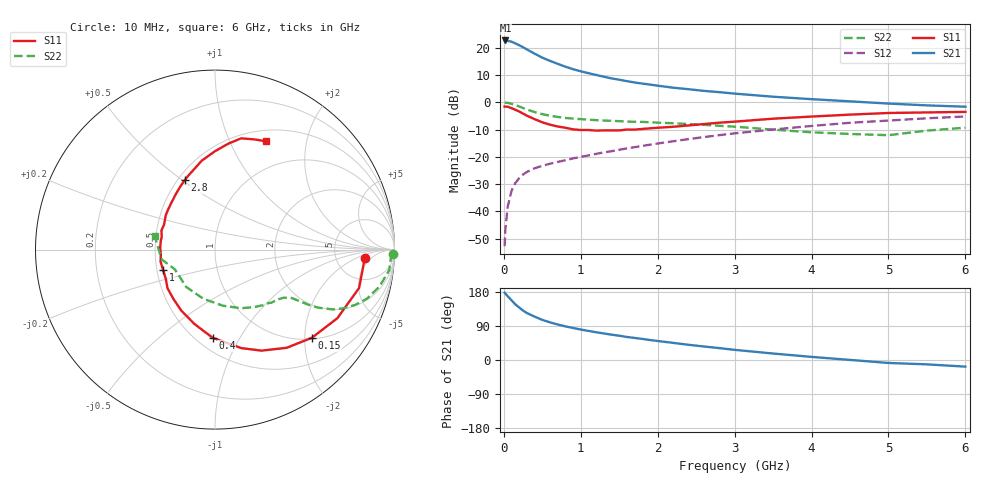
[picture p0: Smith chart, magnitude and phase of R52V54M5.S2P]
! SIEMENS Small Signal Semiconductors
! BFR183
! Si NPN RF Bipolar Junction Transistor in SOT23
! VCE = 2.5 V  IC = 4.5 mA
! Common Emitter S-Parameters:  May  1996
# GHz  S  MA  R  50
!  f  S11  S21  S12  S22
! GHz  MAG  ANG  MAG  ANG  MAG  ANG  MAG  ANG
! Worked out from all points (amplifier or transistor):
!   36 points, 10 MHz to 6 GHz, reference 50 ohm
!   highest |S21| = 22.7 dB at 20 MHz (marker M1)
!   |S21| within 3 dB of that: start of sweep to 281.9 MHz
!   unconditionally stable (mu >= 1): 1.077 GHz to 2.656 GHz
!   at 250 MHz: K = 0.39, MSG = 23.3 dB, |S12| = -26.4 dB
!   at 1.4 GHz: K = 1.06, MAG = 11.8 dB, |S12| = -17.9 dB
!   at 6 GHz: K = 0.89, MSG = 1.8 dB, |S12| = -5.2 dB
!   S11 on the Smith chart (normalised r, x): 10 MHz: 10, -3; 150 MHz: 1.03, -2.17; 400 MHz: 0.60, -0.77; 1 GHz: 0.54, -0.14; 2.8 GHz: 0.54, +0.51; 6 GHz: 0.63, +1.38
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0.01  0.8343 -3.1  13.59 177.8  0.0023 86.5  0.9919 -1.3
0.02  0.8317 -5.9  13.62 175.2  0.0047 86.4  0.981 -2.7
0.05  0.8308 -14.9  13.4 168.4  0.0122 81.5  0.9776 -6.7
0.1  0.7815 -29.3  12.92 157.5  0.0238 75.7  0.9398 -12.6
0.15  0.7298 -42.3  12.02 146.7  0.0332 69.2  0.8898 -17.9
0.2  0.6772 -53.9  11.13 138.4  0.0407 65.0  0.8386 -21.6
0.25  0.6196 -65.3  10.23 130.4  0.0476 60.8  0.7842 -24.7
0.3  0.5682 -75.0  9.326 123.9  0.0529 58.6  0.7364 -26.9
0.4  0.4912 -91.6  7.794 114.4  0.0617 55.1  0.6623 -29.3
0.5  0.4294 -105.6  6.597 105.9  0.0685 54.1  0.6073 -30.5
0.6  0.3885 -118.8  5.755 99.3  0.0748 53.9  0.567 -31.1
0.7  0.3602 -129.8  5.075 93.7  0.0805 54.2  0.5396 -31.6
0.8  0.3411 -140.9  4.498 88.8  0.0867 54.4  0.5166 -32.0
1  0.3107 -158.6  3.7 80.4  0.0998 55.5  0.4914 -32.9
1.1  0.3106 -167.3  3.422 76.8  0.1061 56.1  0.4802 -33.9
1.6  0.3169 160.3  2.44 60.8  0.1429 57.7  0.4432 -38.9
2.2  0.3555 133.5  1.853 45.2  0.1929 56.4  0.4133 -48.1
2.8  0.4228 113.5  1.535 31.4  0.2495 52.5  0.3709 -60.7
3.5  0.5007 98.5  1.266 17.1  0.317 45.5  0.3156 -82.0
4.5  0.5944 82.9  1.042 0.2  0.4211 33.4  0.2627 -127.7
5.5  0.6524 70.2  0.878 -11.5  0.5092 20.7  0.3026 -169.7
6  0.6671 64.8  0.83 -17.5  0.5497 12.5  0.3427 167.6
